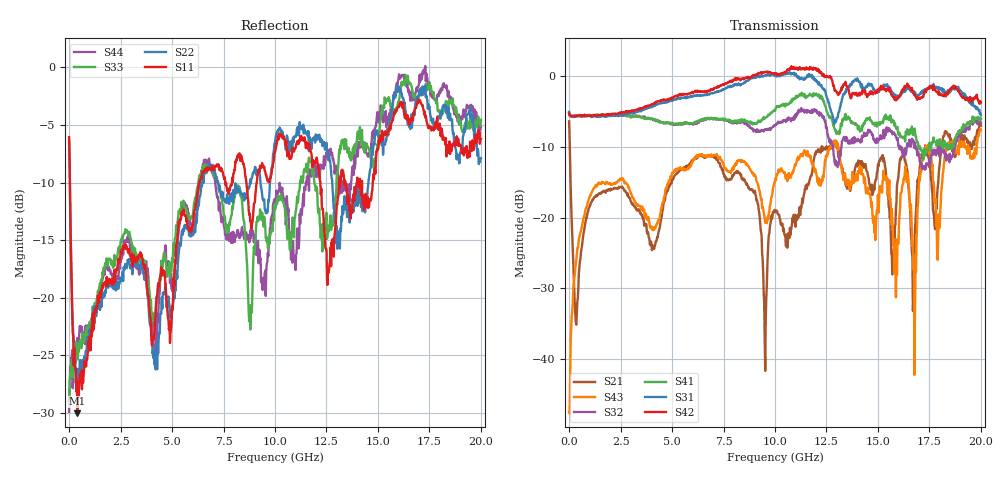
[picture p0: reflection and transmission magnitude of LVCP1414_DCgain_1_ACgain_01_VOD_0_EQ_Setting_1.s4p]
!Agilent Technologies,N5230A,MY46400459,A.07.50.48
!Agilent N5230A: A.07.50.48
!Date: Tuesday, April 17, 2012 18:45:23
!Correction: S11(Full 4 Port(1,2,3,4))
!S12(Full 4 Port(1,2,3,4))
!S13(Full 4 Port(1,2,3,4))
!S14(Full 4 Port(1,2,3,4))
!S21(Full 4 Port(1,2,3,4))
!S22(Full 4 Port(1,2,3,4))
!S23(Full 4 Port(1,2,3,4))
!S24(Full 4 Port(1,2,3,4))
!S31(Full 4 Port(1,2,3,4))
!S32(Full 4 Port(1,2,3,4))
!S33(Full 4 Port(1,2,3,4))
!S34(Full 4 Port(1,2,3,4))
!S41(Full 4 Port(1,2,3,4))
!S42(Full 4 Port(1,2,3,4))
!S43(Full 4 Port(1,2,3,4))
!S44(Full 4 Port(1,2,3,4))
!S4P File: Measurements: <S11,S12,S13,S14>,
!<S21,S22,S23,S24>,
!<S31,S32,S33,S34>,
!<S41,S42,S43,S44>:
# Hz S  dB  R 50
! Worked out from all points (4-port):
!   801 points, 300 kHz to 20 GHz, reference 50 ohm
!   strongest paths, dB at 300 kHz, 5 GHz, 10 GHz, 15 GHz, 20 GHz:
!     S42: -5.3, -3.1, 0.2, -2.0, -3.7
!     S31: -5.1, -3.5, -0.1, -2.3, -5.6
!     S41: -5.2, -6.6, -5.0, -6.7, -6.1
!     S32: -5.3, -6.8, -7.0, -9.4, -6.7
!     S43: -47.4, -13.7, -15.0, -16.8, -7.7
!     S21: -6.4, -14.6, -19.2, -12.5, -7.0
!   lowest |S11| = -30.0 dB at 400.3 MHz (marker M1), VSWR 1.06, Z = 53 + j1.34 ohm
!   |S11| at or under -10 dB: 37.32 MHz to 6.311 GHz (6.273 GHz wide, 198 % of centre); 12.2 GHz to 13.1 GHz (901.7 MHz wide, 7.13 % of centre); 13.42 GHz to 13.99 GHz (561.7 MHz wide, 4.1 % of centre)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
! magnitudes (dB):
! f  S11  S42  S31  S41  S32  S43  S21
! 300 kHz  -6.1  -5.3  -5.1  -5.2  -5.3  -47.4  -6.4
! 400.3 MHz  -30.0  -5.7  -5.6  -5.6  -5.6  -24.3  -31.8
! 10.08 GHz  -6.7  0.3  0.1  -4.3  -6.8  -13.9  -19.0
! 12.7 GHz  -15.6  -0.3  -4.8  -5.8  -9.5  -10.1  -10.3
! 16.8 GHz  -3.5  -2.6  -2.4  -7.9  -9.5  -32.7  -21.6
! 17.3 GHz  -4.4  -2.0  -2.1  -11.2  -12.9  -10.0  -9.8
! 20 GHz  -6.2  -3.7  -5.6  -6.1  -6.7  -7.7  -7.0
